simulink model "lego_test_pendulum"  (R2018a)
settings: Solver=VariableStepAuto  StartTime=0.0  StopTime=3  RelTol=1e-3
model workspace: external: MATLAB File (data not in the file)
undefined symbols (not defined in the file): cm, deg, kg, m, mm, N, rad, s, smiData, X, Y, Z
libraries: sm_lib x60, nesl_utility x3, simulink_extras x2
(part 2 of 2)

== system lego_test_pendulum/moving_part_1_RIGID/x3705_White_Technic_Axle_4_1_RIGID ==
  ReferenceFrame : sm_lib/Frames and Transforms/Reference Frame
  Solid : sm_lib/Body Elements/Solid  InertiaType=Custom  Mass=smiData.Solid(2).mass  MassUnits=kg  CenterOfMass=smiData.Solid(2).CoM  CenterOfMassUnits=mm  MomentsOfInertia=smiData.Solid(2).MoI  MomentsOfInertiaUnits=kg*mm^2  ProductsOfInertia=smiData.Solid(2).PoI  ProductsOfInertiaUnits=kg*mm^2  DensityBased=on  Density=1000  DensityUnits=kg/m^3  DoExposeReferenceFrame=on  SerializedFrames=<Frames/>  GraphicType=FromGeometry  MarkerShape=Sphere  MarkerSize=10  GraphicVisPropType=SimpleVisualProperties  GraphicDiffuseColor=smiData.Solid(2).color  GraphicSpecularColor=[0.5 0.5 0.5 1.0]  GraphicAmbientColor=[0.15 0.15 0.15 1.0]  GraphicEmissiveColor=[0.0 0.0 0.0 1.0]  GraphicShininess=75  GraphicOpacity=smiData.Solid(2).opacity  GeometryShape=FromFile  RectangleSize=[1 1]  RectangleSizeUnits=m  BrickDimensions=[1 1 1]  BrickDimensionUnits=m  CylinderRadius=1  CylinderRadiusUnits=m  CylinderLength=1  CylinderLengthUnits=m  SphereRadius=1  SphereRadiusUnits=m  EllipsoidRadii=[1 1 1]  EllipsoidRadiiUnits=m  ExtrusionCrossSection=[1 1; -1 1; -1 -1; 1 -1]  ExtrusionCrossSectionUnits=m  ExtrusionLength=1  ExtrusionLengthUnits=m  PolygonNumSides=3  PolygonOuterRadius=1  PolygonOuterRadiusUnits=m  ExtGeomFileType=STEP  ExtGeomFileName=3705 White Technic Axle 4_Predeterminado_sldprt.STEP  ExtGeomFileUnits=m  RevolutionCrossSection=[1 1; 1 -1; 2 -1; 2 1]  RevolutionCrossSectionUnits=m  RevolutionExtent=Full  RevolutionAngle=180  RevolutionAngleUnits=deg
  F : PMIOPort  Side=Left
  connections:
  Solid/RConn1 -- ReferenceFrame/RConn1 -- F/RConn1

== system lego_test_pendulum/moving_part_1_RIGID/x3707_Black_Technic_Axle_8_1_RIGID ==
  ReferenceFrame : sm_lib/Frames and Transforms/Reference Frame
  Solid : sm_lib/Body Elements/Solid  InertiaType=Custom  Mass=smiData.Solid(6).mass  MassUnits=kg  CenterOfMass=smiData.Solid(6).CoM  CenterOfMassUnits=mm  MomentsOfInertia=smiData.Solid(6).MoI  MomentsOfInertiaUnits=kg*mm^2  ProductsOfInertia=smiData.Solid(6).PoI  ProductsOfInertiaUnits=kg*mm^2  DensityBased=on  Density=1000  DensityUnits=kg/m^3  DoExposeReferenceFrame=on  SerializedFrames=<Frames/>  GraphicType=FromGeometry  MarkerShape=Sphere  MarkerSize=10  GraphicVisPropType=SimpleVisualProperties  GraphicDiffuseColor=smiData.Solid(6).color  GraphicSpecularColor=[0.5 0.5 0.5 1.0]  GraphicAmbientColor=[0.15 0.15 0.15 1.0]  GraphicEmissiveColor=[0.0 0.0 0.0 1.0]  GraphicShininess=75  GraphicOpacity=smiData.Solid(6).opacity  GeometryShape=FromFile  RectangleSize=[1 1]  RectangleSizeUnits=m  BrickDimensions=[1 1 1]  BrickDimensionUnits=m  CylinderRadius=1  CylinderRadiusUnits=m  CylinderLength=1  CylinderLengthUnits=m  SphereRadius=1  SphereRadiusUnits=m  EllipsoidRadii=[1 1 1]  EllipsoidRadiiUnits=m  ExtrusionCrossSection=[1 1; -1 1; -1 -1; 1 -1]  ExtrusionCrossSectionUnits=m  ExtrusionLength=1  ExtrusionLengthUnits=m  PolygonNumSides=3  PolygonOuterRadius=1  PolygonOuterRadiusUnits=m  ExtGeomFileType=STEP  ExtGeomFileName=3707 Black Technic Axle 8_Predeterminado_sldprt.STEP  ExtGeomFileUnits=m  RevolutionCrossSection=[1 1; 1 -1; 2 -1; 2 1]  RevolutionCrossSectionUnits=m  RevolutionExtent=Full  RevolutionAngle=180  RevolutionAngleUnits=deg
  F : PMIOPort  Side=Left
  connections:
  Solid/RConn1 -- ReferenceFrame/RConn1 -- F/RConn1

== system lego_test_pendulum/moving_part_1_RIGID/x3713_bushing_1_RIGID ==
  ReferenceFrame : sm_lib/Frames and Transforms/Reference Frame
  Solid : sm_lib/Body Elements/Solid  InertiaType=Custom  Mass=smiData.Solid(5).mass  MassUnits=kg  CenterOfMass=smiData.Solid(5).CoM  CenterOfMassUnits=cm  MomentsOfInertia=smiData.Solid(5).MoI  MomentsOfInertiaUnits=kg*cm^2  ProductsOfInertia=smiData.Solid(5).PoI  ProductsOfInertiaUnits=kg*cm^2  DensityBased=on  Density=1000  DensityUnits=kg/m^3  DoExposeReferenceFrame=on  SerializedFrames=<Frames/>  GraphicType=FromGeometry  MarkerShape=Sphere  MarkerSize=10  GraphicVisPropType=SimpleVisualProperties  GraphicDiffuseColor=smiData.Solid(5).color  GraphicSpecularColor=[0.5 0.5 0.5 1.0]  GraphicAmbientColor=[0.15 0.15 0.15 1.0]  GraphicEmissiveColor=[0.0 0.0 0.0 1.0]  GraphicShininess=75  GraphicOpacity=smiData.Solid(5).opacity  GeometryShape=FromFile  RectangleSize=[1 1]  RectangleSizeUnits=m  BrickDimensions=[1 1 1]  BrickDimensionUnits=m  CylinderRadius=1  CylinderRadiusUnits=m  CylinderLength=1  CylinderLengthUnits=m  SphereRadius=1  SphereRadiusUnits=m  EllipsoidRadii=[1 1 1]  EllipsoidRadiiUnits=m  ExtrusionCrossSection=[1 1; -1 1; -1 -1; 1 -1]  ExtrusionCrossSectionUnits=m  ExtrusionLength=1  ExtrusionLengthUnits=m  PolygonNumSides=3  PolygonOuterRadius=1  PolygonOuterRadiusUnits=m  ExtGeomFileType=STEP  ExtGeomFileName=3713 - bushing_Default_sldprt.STEP  ExtGeomFileUnits=m  RevolutionCrossSection=[1 1; 1 -1; 2 -1; 2 1]  RevolutionCrossSectionUnits=m  RevolutionExtent=Full  RevolutionAngle=180  RevolutionAngleUnits=deg
  F : PMIOPort  Side=Left
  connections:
  Solid/RConn1 -- ReferenceFrame/RConn1 -- F/RConn1
